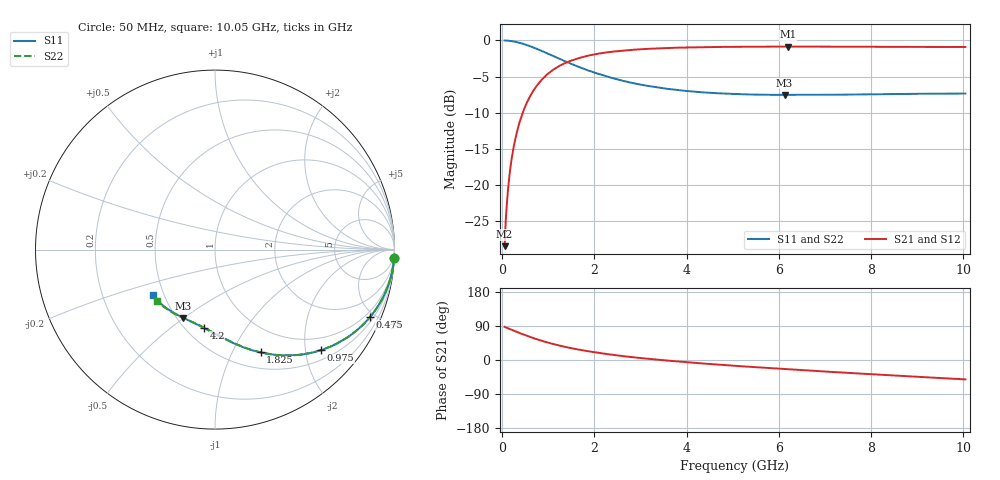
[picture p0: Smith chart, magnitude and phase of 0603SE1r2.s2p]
! AVX Thin Film Operation		Date: August 2001
! Description: Accu-P® Series, Thin Film, SMD, RF Capacitor
! Part Number: 06035J1R2ABT
! 50 MHz  -  10.05 GHz
! Serial Measurements
# mhz S db R 50
!	S11		S21		S12		S22
!	dB	Phase	dB	Phase	dB	Phase	dB	Phase
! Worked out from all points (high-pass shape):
!   401 points, 50 MHz to 10.05 GHz, reference 50 ohm
!   highest |S21| = -0.86 dB at 6.2 GHz (marker M1); lowest = -28.5 dB at 50 MHz (marker M2)
!   |S21| within 3 dB of the highest: 1.159 GHz to end of sweep
!   lowest |S11| = -7.6 dB at 6.125 GHz (marker M3), VSWR 2.44, Z = 26.9 - j24.9 ohm
!   |S11| at or under -10 dB: nowhere
!   |S22| runs from -7.5 to 0.0 dB; largest |S21 - S12| = 0
!   S11 on the Smith chart (normalised r, x): 50 MHz: 1, -45; 475 MHz: 0.71, -4.71; 975 MHz: 0.70, -2.32; 1.825 GHz: 0.69, -1.29; 4.2 GHz: 0.61, -0.66; 10.05 GHz: 0.44, -0.27
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50  -0.01 -2.6  -28.50 87.4  -28.50 87.4  -0.01 -2.6
75  -0.01 -3.9  -24.93 86.1  -24.93 86.1  -0.01 -3.9
125  -0.04 -6.4  -20.59 83.6  -20.59 83.6  -0.04 -6.4
150  -0.06 -7.7  -19.01 82.3  -19.01 82.3  -0.06 -7.7
225  -0.12 -11.5  -15.56 78.5  -15.56 78.5  -0.12 -11.5
325  -0.25 -16.4  -12.49 73.5  -12.49 73.5  -0.25 -16.4
475  -0.52 -23.5  -9.48 66.5  -9.48 66.5  -0.52 -23.5
700  -1.04 -33.3  -6.71 56.7  -6.71 56.7  -1.04 -33.3
975  -1.79 -43.5  -4.71 46.5  -4.71 46.5  -1.79 -43.5
1350  -2.86 -55.0  -3.18 35.0  -3.18 35.0  -2.86 -55.0
1725  -3.83 -64.1  -2.33 25.9  -2.33 25.9  -3.83 -64.0
1825  -4.07 -66.1  -2.17 23.9  -2.17 23.9  -4.06 -66.0
2175  -4.81 -72.7  -1.75 17.4  -1.75 17.4  -4.81 -72.5
2525  -5.45 -78.5  -1.47 11.6  -1.47 11.6  -5.45 -78.2
3400  -6.54 -89.8  -1.10 0.5  -1.10 0.5  -6.54 -89.1
4200  -7.12 -98.1  -0.95 -7.8  -0.95 -7.8  -7.11 -97.1
5050  -7.42 -106.0  -0.88 -15.4  -0.88 -15.4  -7.41 -104.6
6125  -7.55 -114.9  -0.86 -24.0  -0.86 -24.0  -7.53 -112.9
6200  -7.55 -115.9  -0.86 -24.5  -0.86 -24.5  -7.53 -113.0
6725  -7.55 -119.9  -0.86 -28.5  -0.86 -28.5  -7.53 -116.9
8400  -7.44 -132.2  -0.89 -40.2  -0.89 -40.2  -7.41 -128.2
10050  -7.36 -143.8  -0.91 -51.2  -0.91 -51.2  -7.33 -138.4
